(* Logix 5000 Rung export; software revision 16.04 *)

TYPE ICX35_STATUS :   // ICX35 Status
STRUCT
   RSSI : SINT;   // Current Signal Strength dBm. Range -50 to -125
   Min_RSSI : SINT;   // Signal Strength Minimum(since power on). Range -50 to -125
   Max_RSSI : SINT;   // Signal Strength Maximum(since power on). Range -50 to -125
   Cell_Net_State : SINT;   // Status of the connection to the Cellular Network. 0: Disconnect, 1: Connecting, 2: Connected
   MAC_Address : SINT[6];   // MAC ID of ICX35
   WAN_IP : INT[4];   // Cellular network IP
   Cell_Net_Disconnects : DINT;   // Number of times Modem is disconnected from the cellular network since power on
   LAN_KBytes_Sent : DINT;   // Number Kbytes sent on LAN since power on
   LAN_KBytes_Received : DINT;   // Number of Kbytes received LAN since power on
   WAN_KBytes_Sent : DINT;   // Number of Bytes Sent WAN since power on
   WAN_KBytes_Received : DINT;   // Number of bytes received WAN since power on
   SMS_MSGs_Sent : DINT;   // Number of SMS Messages Sent since power on
   SMS_MSGs_Received : DINT;   // Number of SMS Messages Sent since power on
   SMS_MSGs_Rx_Free_Buffer_Counter : DINT;   // Number of free slots in the Rx SMS buffer out of 255 Message slots.
   PowerOnTime_Year : INT;   // Power on time year
   PowerOnTime_Month : INT;   // Power on time month
   PowerOnTime_Day : INT;   // Power on time day
   PowerOnTime_Hour : INT;   // Power on time hour
   PowerOnTime_Minute : INT;   // Power on time minute
   PowerOnTime_Second : INT;   // Power on time second
   Link_Time_Days : DINT;   // Link Time: Days of Cellular Connection.
   Link_Time_Hours : DINT;   // Link Time: Hours of Cellular Connection.
   Link_Time_Minutes : INT;   // Link Time: Minutes of Cellular Connection.
   Link_Time_Seconds : INT;   // Link Time: Seconds of Cellular Connection.
   Data_Usage_Current_Month : DINT;   // Data usage of current month in KB.
   Data_Usage_Previous_Month : DINT;   // Data usage of last month in KB.
   Data_Usage_Current_Day : DINT;   // Data usage for today in KB.
   Data_Usage_Previous_Day : DINT;   // Data usage of yesterday in KB.
   FW_Version : SINT[24];   // Firmware Version for the Gateway
   Phone_Number : SINT[18];   // Cellular phone number
   IMEI : SINT[20];   // IMEI number
END_STRUCT
END_TYPE

TYPE ICX35_ModuleDef :   // Main ICX35 definition
STRUCT
   CONTROL : ICX35_CONTROL;   // Trigger bits used to request functions from ICX35
   STATUS : ICX35_STATUS;   // ICX35 status
   SMS : ICX35_SMS;   // SMS send and receive functions
   UTIL : ICX35_UTIL;   // Tags used for internal processing - do not update the values
END_STRUCT
END_TYPE

TYPE ICX35_CONTROL :   // Contains trigger bits for the functions supported by the ICX35. Bit should be set as 1 to trigger request and AOI will automa
STRUCT
   Get_Status : BOOL;   // Reads status data from ICX35
   Reset_Status : BOOL;   // Resets status counters from ICX35
   Write_SMS : BOOL;   // Sends SMS message to ICX35
   Read_SMS : BOOL;   // Reads SMS message from ICX35
   Clear_SMS : BOOL;   // Clears all SMS from ICX35
   Reboot : BOOL;   // Reboot ICX35
END_STRUCT
END_TYPE

TYPE ICX35_UTIL :   // Internal tag used for internal ladder processing. Not to be updated by user application
STRUCT
   Status : SINT[149];   // Receives Raw Status Data from the Gateway
   SMSwrite : SINT[284];   // Text Messages (SMS) to be sent.
   SMSread : SINT[216];   // Text Messages that are read.
   SMSwritemsgstat : BOOL;   // SMS Write MSG instruction status.
   SMSreadmsgstat : BOOL;   // SMS Read MSG instruction status.
   ResetStatus : SINT;   // Reset speceific Status counters.
   Clear_SMS : SINT;   // Clear SMS Messages
   Reboot : SINT;   // Reboot ICX35 Gateway
END_STRUCT
END_TYPE

TYPE ICX35_SMS_Read :   // SMS data read from ICX35
STRUCT
   Date_Time : SINT[18];   // DateTime Stamp for received SMS text. MM/DD/YY HH:MM:SS
   Time_Zone : SINT[6];   // UTC =/- TZ
   Phone_Number : SINT[24];   // full number including prefixes country code etc..
   Message : SINT[160];   // Received the message text
END_STRUCT
END_TYPE

TYPE ICX35_SMS_Write :   // SMS data written to ICX35
STRUCT
   Message : LSTRING;
   Phone_Count : INT;   // Quantity of phone numbers that the SMS will be sent to. 5 is the limit.
   Phone_Number_1 : SINT[24];   // full number including prefixes country code (example +16613334455)
   Phone_Number_2 : SINT[24];   // full number including prefixes country code
   Phone_Number_3 : SINT[24];   // full number including prefixes country code
   Phone_Number_4 : SINT[24];   // full number including prefixes country code
   Phone_Number_5 : SINT[24];   // full number including prefixes country code
END_STRUCT
END_TYPE

TYPE ICX35_SMS :   // Stores main SMS functions
STRUCT
   READ : ICX35_SMS_Read;   // Reads SMS data from ICX35
   WRITE : ICX35_SMS_Write;   // Writes SMS message to ICX35
END_STRUCT
END_TYPE

TYPE LSTRING :   // string type
STRUCT
   LEN : DINT;
   DATA : SINT[160];
END_STRUCT
END_TYPE

ADD_ON_INSTRUCTION AOI_ICX35   (* revision 1.8 *)
// Add-On Instruction for ICX35 Industrial Cellular Gateway
// Revision note:
// 1.8    2018/06/14.
// This Revision is compatible with ICX35 firmware version 1.4 and later.
VAR_IN_OUT
   ICX35 : ICX35_ModuleDef; {required}
   ICX35_MSG_GET_STATUS : MESSAGE; {required}
   ICX35_MSG_READ_SMS : MESSAGE; {required}
   ICX35_MSG_RESET_STATUS : MESSAGE; {required}
   ICX35_MSG_WRITE_SMS : MESSAGE; {required}
   ICX35_MSG_CLEAR_SMS : MESSAGE; {required}
   ICX35_MSG_REBOOT : MESSAGE; {required}
END_VAR

ROUTINE Logic   (* ladder *)
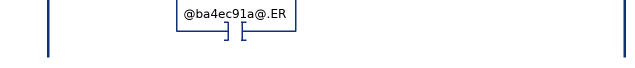
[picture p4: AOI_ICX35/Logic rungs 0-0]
   0: XIC(@2c793ec3@.CONTROL.Get_Status)[MSG(@ba4ec91a@) ,XIC(@ba4ec91a@.DN) [COP(@2c793ec3@.UTIL.Status[0],@2c793ec3@.STATUS.RSSI,4) ,COP(@2c793ec3@.UTIL.Status[4],@2c793ec3@.STATUS.MAC_Address[0],6) ,MVM(0,65280,@2c793ec3@.STATUS.WAN_IP[0]) ,MVM(@2c793ec3@.UTIL.Status[10],255,@2c793ec3@.STATUS.WAN_IP[0]) ,MVM(0,65280,@2c793ec3@.STATUS.WAN_IP[1]) ,MVM(@2c793ec3@.UTIL.Status[11],255,@2c793ec3@.STATUS.WAN_IP[1]) ,MVM(0,65280,@2c793ec3@.STATUS.WAN_IP[2]) ,MVM(@2c793ec3@.UTIL.Status[12],255,@2c793ec3@.STATUS.WAN_IP[2]) ,MVM(0,65280,@2c793ec3@.STATUS.WAN_IP[3]) ,MVM(@2c793ec3@.UTIL.Status[13],255,@2c793ec3@.STATUS.WAN_IP[3]) ,COP(@2c793ec3@.UTIL.Status[14],@2c793ec3@.STATUS.Cell_Net_Disconnects,1) ,COP(@2c793ec3@.UTIL.Status[18],@2c793ec3@.STATUS.LAN_KBytes_Sent,1) ,COP(@2c793ec3@.UTIL.Status[22],@2c793ec3@.STATUS.LAN_KBytes_Received,1) ,COP(@2c793ec3@.UTIL.Status[26],@2c793ec3@.STATUS.WAN_KBytes_Sent,1) ,COP(@2c793ec3@.UTIL.Status[30],@2c793ec3@.STATUS.WAN_KBytes_Received,1) ,COP(@2c793ec3@.UTIL.Status[34],@2c793ec3@.STATUS.SMS_MSGs_Sent,1) ,COP(@2c793ec3@.UTIL.Status[38],@2c793ec3@.STATUS.SMS_MSGs_Received,1) ,COP(@2c793ec3@.UTIL.Status[42],@2c793ec3@.STATUS.SMS_MSGs_Rx_Free_Buffer_Counter,1) ,COP(@2c793ec3@.UTIL.Status[46],@2c793ec3@.STATUS.PowerOnTime_Year,1) ,COP(@2c793ec3@.UTIL.Status[48],@2c793ec3@.STATUS.PowerOnTime_Month,1) ,COP(@2c793ec3@.UTIL.Status[50],@2c793ec3@.STATUS.PowerOnTime_Day,1) ,COP(@2c793ec3@.UTIL.Status[52],@2c793ec3@.STATUS.PowerOnTime_Hour,1) ,COP(@2c793ec3@.UTIL.Status[54],@2c793ec3@.STATUS.PowerOnTime_Minute,1) ,COP(@2c793ec3@.UTIL.Status[56],@2c793ec3@.STATUS.PowerOnTime_Second,1) ,COP(@2c793ec3@.UTIL.Status[58],@2c793ec3@.STATUS.Link_Time_Days,1) ,COP(@2c793ec3@.UTIL.Status[62],@2c793ec3@.STATUS.Link_Time_Hours,1) ,COP(@2c793ec3@.UTIL.Status[66],@2c793ec3@.STATUS.Link_Time_Minutes,1) ,COP(@2c793ec3@.UTIL.Status[68],@2c793ec3@.STATUS.Link_Time_Seconds,1) ,COP(@2c793ec3@.UTIL.Status[70],@2c793ec3@.STATUS.Data_Usage_Current_Day,1) ,COP(@2c793ec3@.UTIL.Status[74],@2c793ec3@.STATUS.Data_Usage_Current_Month,1) ,COP(@2c793ec3@.UTIL.Status[78],@2c793ec3@.STATUS.Data_Usage_Previous_Day,1) ,COP(@2c793ec3@.UTIL.Status[82],@2c793ec3@.STATUS.Data_Usage_Previous_Month,1) ,COP(@2c793ec3@.UTIL.Status[86],@2c793ec3@.STATUS.FW_Version[0],24) ,COP(@2c793ec3@.UTIL.Status[110],@2c793ec3@.STATUS.Phone_Number[0],18) ,COP(@2c793ec3@.UTIL.Status[128],@2c793ec3@.STATUS.IMEI[0],20) ] ,[XIC(@ba4ec91a@.DN) ,XIC(@ba4ec91a@.ER) ] OTU(@2c793ec3@.CONTROL.Get_Status) ];
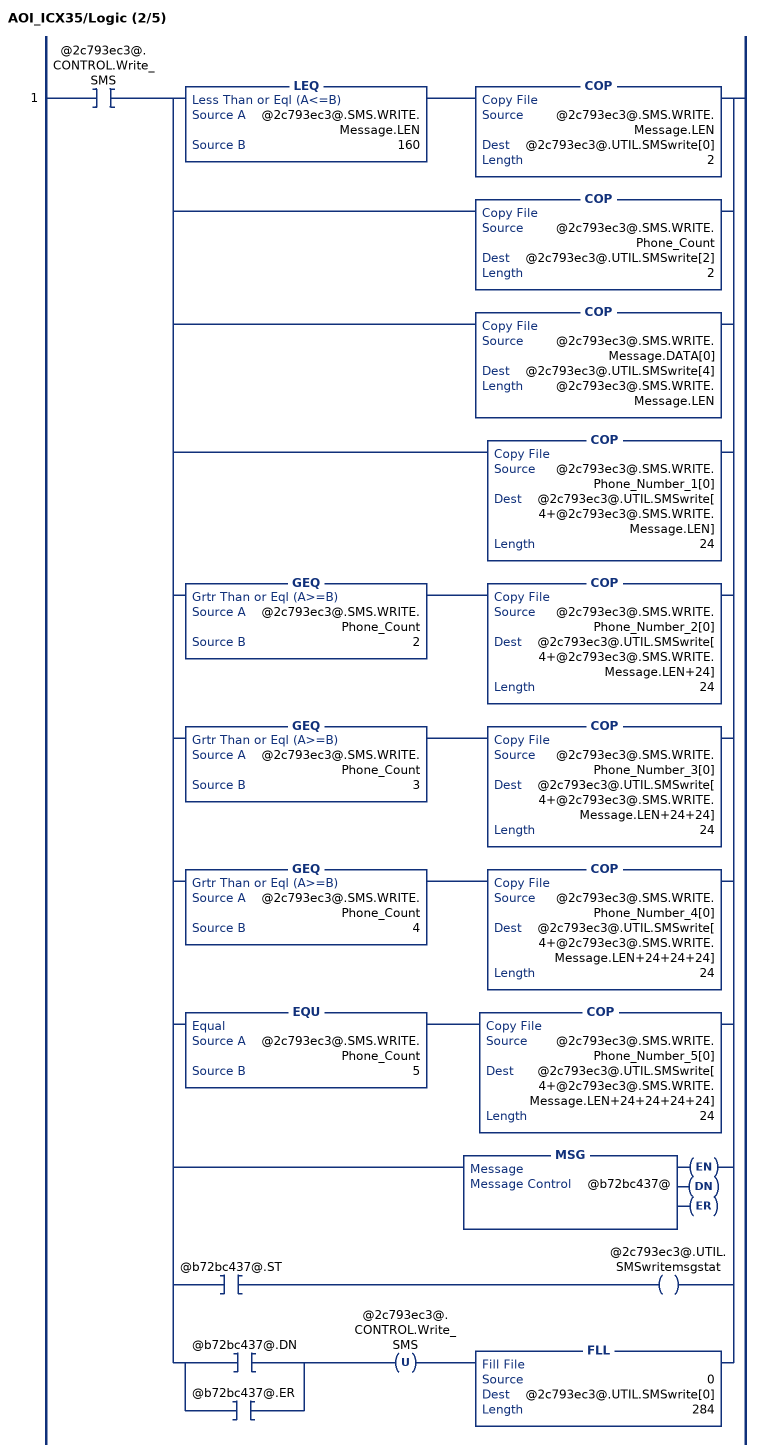
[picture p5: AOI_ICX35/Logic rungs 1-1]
   1: XIC(@2c793ec3@.CONTROL.Write_SMS)[LEQ(@2c793ec3@.SMS.WRITE.Message.LEN,160) COP(@2c793ec3@.SMS.WRITE.Message.LEN,@2c793ec3@.UTIL.SMSwrite[0],2) ,COP(@2c793ec3@.SMS.WRITE.Phone_Count,@2c793ec3@.UTIL.SMSwrite[2],2) ,COP(@2c793ec3@.SMS.WRITE.Message.DATA[0],@2c793ec3@.UTIL.SMSwrite[4],@2c793ec3@.SMS.WRITE.Message.LEN) ,COP(@2c793ec3@.SMS.WRITE.Phone_Number_1[0],@2c793ec3@.UTIL.SMSwrite[4+@2c793ec3@.SMS.WRITE.Message.LEN],24) ,GEQ(@2c793ec3@.SMS.WRITE.Phone_Count,2) COP(@2c793ec3@.SMS.WRITE.Phone_Number_2[0],@2c793ec3@.UTIL.SMSwrite[4+@2c793ec3@.SMS.WRITE.Message.LEN+24],24) ,GEQ(@2c793ec3@.SMS.WRITE.Phone_Count,3) COP(@2c793ec3@.SMS.WRITE.Phone_Number_3[0],@2c793ec3@.UTIL.SMSwrite[4+@2c793ec3@.SMS.WRITE.Message.LEN+24+24],24) ,GEQ(@2c793ec3@.SMS.WRITE.Phone_Count,4) COP(@2c793ec3@.SMS.WRITE.Phone_Number_4[0],@2c793ec3@.UTIL.SMSwrite[4+@2c793ec3@.SMS.WRITE.Message.LEN+24+24+24],24) ,EQU(@2c793ec3@.SMS.WRITE.Phone_Count,5) COP(@2c793ec3@.SMS.WRITE.Phone_Number_5[0],@2c793ec3@.UTIL.SMSwrite[4+@2c793ec3@.SMS.WRITE.Message.LEN+24+24+24+24],24) ,MSG(@b72bc437@) ,XIC(@b72bc437@.ST) OTE(@2c793ec3@.UTIL.SMSwritemsgstat) ,[XIC(@b72bc437@.DN) ,XIC(@b72bc437@.ER) ] OTU(@2c793ec3@.CONTROL.Write_SMS) FLL(0,@2c793ec3@.UTIL.SMSwrite[0],284) ];
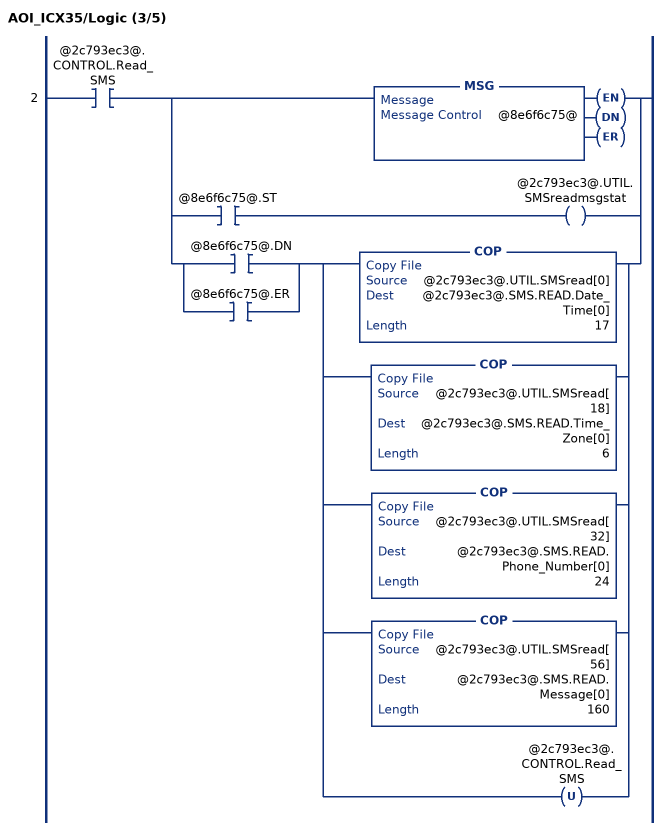
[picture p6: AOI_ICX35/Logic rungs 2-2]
   2: XIC(@2c793ec3@.CONTROL.Read_SMS)[MSG(@8e6f6c75@) ,XIC(@8e6f6c75@.ST) OTE(@2c793ec3@.UTIL.SMSreadmsgstat) ,[XIC(@8e6f6c75@.DN) ,XIC(@8e6f6c75@.ER) ] [COP(@2c793ec3@.UTIL.SMSread[0],@2c793ec3@.SMS.READ.Date_Time[0],17) ,COP(@2c793ec3@.UTIL.SMSread[18],@2c793ec3@.SMS.READ.Time_Zone[0],6) ,COP(@2c793ec3@.UTIL.SMSread[32],@2c793ec3@.SMS.READ.Phone_Number[0],24) ,COP(@2c793ec3@.UTIL.SMSread[56],@2c793ec3@.SMS.READ.Message[0],160) ,OTU(@2c793ec3@.CONTROL.Read_SMS) ] ];
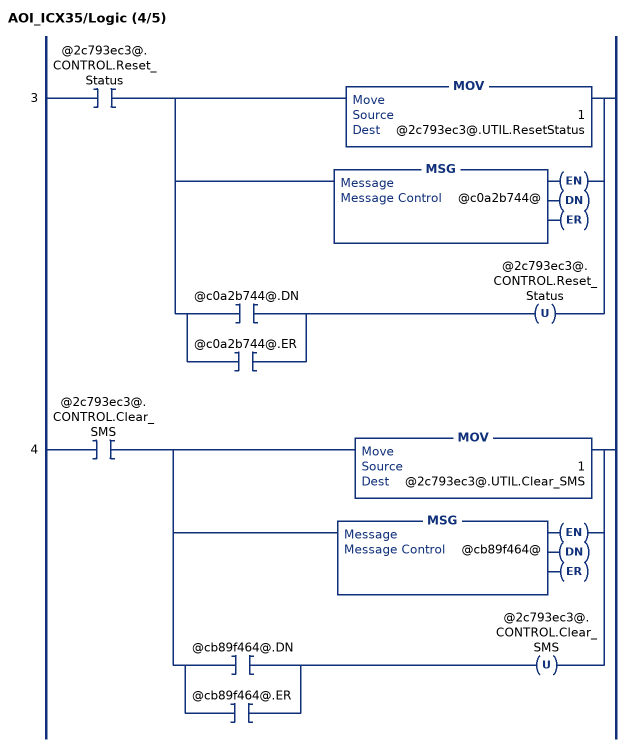
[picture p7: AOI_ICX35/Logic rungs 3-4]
   3: XIC(@2c793ec3@.CONTROL.Reset_Status)[MOV(1,@2c793ec3@.UTIL.ResetStatus) ,MSG(@c0a2b744@) ,[XIC(@c0a2b744@.DN) ,XIC(@c0a2b744@.ER) ] OTU(@2c793ec3@.CONTROL.Reset_Status) ];
   4: XIC(@2c793ec3@.CONTROL.Clear_SMS)[MOV(1,@2c793ec3@.UTIL.Clear_SMS) ,MSG(@cb89f464@) ,[XIC(@cb89f464@.DN) ,XIC(@cb89f464@.ER) ] OTU(@2c793ec3@.CONTROL.Clear_SMS) ];
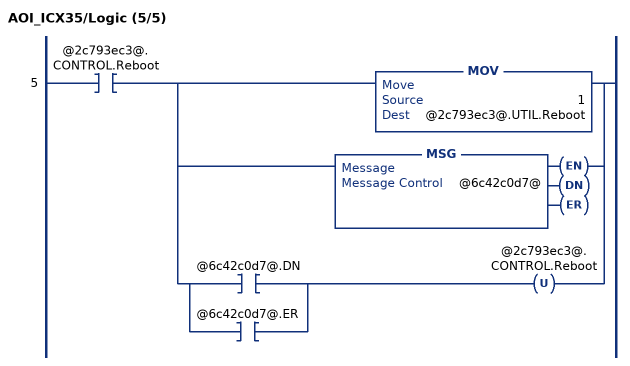
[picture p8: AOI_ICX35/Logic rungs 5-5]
   5: XIC(@2c793ec3@.CONTROL.Reboot)[MOV(1,@2c793ec3@.UTIL.Reboot) ,MSG(@6c42c0d7@) ,[XIC(@6c42c0d7@.DN) ,XIC(@6c42c0d7@.ER) ] OTU(@2c793ec3@.CONTROL.Reboot) ];
END_ROUTINE
END_ADD_ON_INSTRUCTION

VAR_GLOBAL   (* controller tags *)
   ICX35_MSG_RESET_STATUS : MESSAGE;
        MessageParameters(MessageType := CIP Generic, RequestedLength := 1, ConnectedFlag := 2, ConnectionPath := ICX35, ServiceCode := 16#0010, ObjectType := 16#00a2, TargetObject := 1, AttributeNumber := 16#0001, LocalElement := ICX35.UTIL.ResetStatus)
   ICX35_MSG_WRITE_SMS : MESSAGE;
        MessageParameters(MessageType := CIP Generic, RequestedLength := 284, ConnectedFlag := 2, ConnectionPath := ICX35, ServiceCode := 16#0002, ObjectType := 16#00a4, TargetObject := 1, LocalElement := ICX35.UTIL.SMSwrite[0], DestinationTag := ICX35.UTIL.SMSwrite[0])
   ICX35_MSG_READ_SMS : MESSAGE;
        MessageParameters(MessageType := CIP Generic, RequestedLength := 216, ConnectedFlag := 2, ConnectionPath := ICX35, ServiceCode := 16#0001, ObjectType := 16#00a6, TargetObject := 1, LocalElement := ICX35.UTIL.SMSread[0], DestinationTag := ICX35.UTIL.SMSread[0])
   ICX35_MSG_GET_STATUS : MESSAGE;
        MessageParameters(MessageType := CIP Generic, RequestedLength := 144, ConnectedFlag := 2, ConnectionPath := ICX35, ServiceCode := 16#0001, ObjectType := 16#00a1, TargetObject := 1, LocalElement := ICX35.UTIL.Status[0], DestinationTag := ICX35.UTIL.Status[0])
   ICX35 : ICX35_ModuleDef;
   ICX35_MSG_SMS_CLEAR : MESSAGE;
        MessageParameters(MessageType := CIP Generic, RequestedLength := 1, ConnectedFlag := 2, ConnectionPath := ICX35, ServiceCode := 16#0010, ObjectType := 16#00a7, TargetObject := 1, AttributeNumber := 16#0001, LocalElement := ICX35.UTIL.Clear_SMS)
   ICX35_MSG_MOD_REBOOT : MESSAGE;
        MessageParameters(MessageType := CIP Generic, RequestedLength := 1, ConnectedFlag := 2, ConnectionPath := ICX35, ServiceCode := 16#0010, ObjectType := 16#00a8, TargetObject := 1, AttributeNumber := 16#0001, LocalElement := ICX35.UTIL.Reboot)
   AOI_ICX35 : AOI_ICX35;
END_VAR

PROGRAM MainProgram

ROUTINE MainRoutine   (* ladder *)
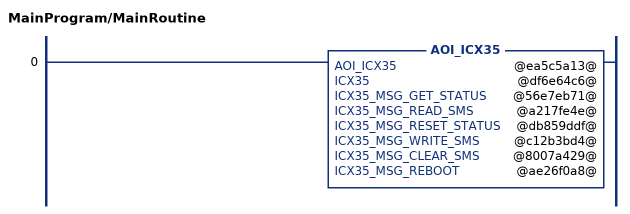
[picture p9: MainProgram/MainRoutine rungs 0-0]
   0: AOI_ICX35(@ea5c5a13@,@df6e64c6@,@56e7eb71@,@a217fe4e@,@db859ddf@,@c12b3bd4@,@8007a429@,@ae26f0a8@);
END_ROUTINE
END_PROGRAM
